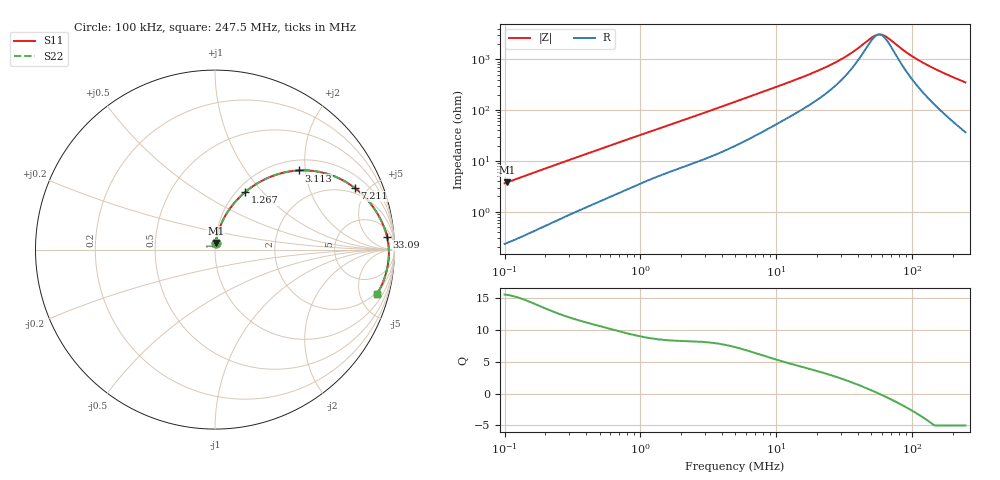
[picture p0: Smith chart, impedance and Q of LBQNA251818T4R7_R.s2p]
! LBQNA251818T4R7_R  S-PARAMETER MODEL  ( General Type )
! Model Generated by TAIYO YUDEN Corporation (http://www.ty-top.com)
! Version 1.0
! TAIYO YUDEN Control No. 191025NI43SB-FBB
! Copyright(c) 2019 TAIYO YUDEN CO.,LTD. All Rights Reserved.
! Product Description (link to TY-COMPAS)
! https://ds.yuden.co.jp/TYCOMPAS/or/detail?pn=LBQNA251818T4R7MR&u=M
! Products Name : Inductors
! Characteristics :
!  Inductance : 4.7 uH , SRF(min) : 46 MHz , DC Resistance(max) : 0.13 Ohm
!  Rated Current : Saturation :310 mA , Temp Rise : 820 mA (20 degC)
!  Case Size : 2.5 x 1.8 / 0.098 x 0.071 [mm/inch] , Thickness : 1.8 / 0.071 [mm/inch]
!  (Conditions: Temperature = 25 degC , DC Bias Current/Voltage = 0A / 0V)
! External Node Assignments :
!  1  o---GGG---o  2
! GND o---------o GND
! Frequency Range : 0.1MHz  -  247.502633MHz  [ 402 STEP ]
# MHz S RI R 50
! Freq[MHz].  S11 Real  S11 Imag  S21 Real  S21 Imag  S12 Real  S12 Imag  S22 Real  S22 Imag
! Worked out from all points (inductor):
!   401 points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, 100 kHz to 247.5 MHz, reference 50 ohm
!   read as one part in series: L = 5.74 uH near 104 kHz
!   highest Q = 15.6 at 104 kHz (marker M1), where L = 5.77 uH
!   self-resonance near 57.22 MHz
!   S11 on the Smith chart (normalised r, x): 100 kHz: 1.00, +0.07; 1.267 MHz: 1.09, +0.80; 3.113 MHz: 1.23, +1.85; 7.211 MHz: 1.65, +4.12; 33.09 MHz: 11, +21; 247.5 MHz: 1.74, -7.00
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0.1  0.00362 0.036  0.9964 -0.036  0.9964 -0.036  0.00362 0.036
0.103984  0.00382 0.0374  0.9962 -0.0374  0.9962 -0.0374  0.00382 0.0374
0.37019  0.0265 0.1227  0.9735 -0.1227  0.9735 -0.1227  0.0265 0.1227
0.733437  0.0761 0.2185  0.9239 -0.2185  0.9239 -0.2185  0.0761 0.2185
1.267399  0.1673 0.3198  0.8327 -0.3198  0.8327 -0.3198  0.1673 0.3198
1.370406  0.1857 0.3347  0.8143 -0.3347  0.8143 -0.3347  0.1857 0.3347
2.025481  0.3012 0.4024  0.6988 -0.4024  0.6988 -0.4024  0.3012 0.4024
3.112971  0.469 0.4411  0.531 -0.4411  0.531 -0.4411  0.469 0.4411
4.974964  0.6603 0.4103  0.3397 -0.4103  0.3397 -0.4103  0.6603 0.4103
7.210825  0.7791 0.3432  0.2209 -0.3432  0.2209 -0.3432  0.7791 0.3432
11.08235  0.8685 0.2536  0.1315 -0.2536  0.1315 -0.2536  0.8685 0.2536
18.41681  0.9269 0.1597  0.0731 -0.1597  0.0731 -0.1597  0.9269 0.1597
25.17432  0.9474 0.1104  0.0526 -0.1104  0.0526 -0.1104  0.9474 0.1104
33.09276  0.9588 0.0715  0.0412 -0.0715  0.0412 -0.0715  0.9588 0.0715
53.93017  0.9683 0.00759  0.0317 -0.00759  0.0317 -0.00759  0.9683 0.00759
57.1852  0.9687 8.81e-05  0.0313 -8.81e-05  0.0313 -8.81e-05  0.9687 8.81e-05
60.63669  0.9689 -0.00744  0.0311 0.00744  0.0311 0.00744  0.9689 -0.00744
68.1772  0.9689 -0.0227  0.0311 0.0227  0.0311 0.0227  0.9689 -0.0227
91.38994  0.9662 -0.0626  0.0338 0.0626  0.0338 0.0626  0.9662 -0.0626
117.8121  0.9601 -0.1009  0.0399 0.1009  0.0399 0.1009  0.9601 -0.1009
167.456  0.9428 -0.1631  0.0572 0.1631  0.0572 0.1631  0.9428 -0.1631
247.5026  0.9032 -0.2478  0.0968 0.2478  0.0968 0.2478  0.9032 -0.2478
